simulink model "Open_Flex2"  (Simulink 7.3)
settings: Solver=ode4  StartTime=0.0  StopTime=20  RelTol=1e-3
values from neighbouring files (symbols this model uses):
  Ts = 0.04    [run.m]    (also in z2s_transf.m)
undefined symbols (not defined in the file or in its folder): Alfc, Apfc, Azpl, Blfc, Bpfc, Bzpl, Clfc, Cpfc, Czpl, Dlfc, Dpfc, Dzpl, TVC

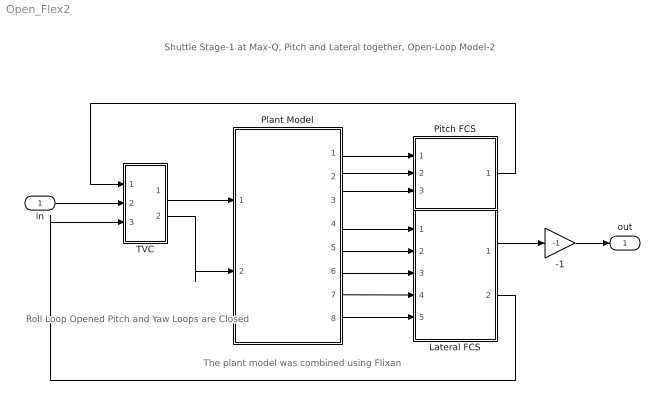
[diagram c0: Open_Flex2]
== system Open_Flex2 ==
  note: Shuttle Stage-1 at Max-Q, Pitch and Lateral together, Open-Loop Model-2
  note: Roll Loop Opened Pitch and Yaw Loops are Closed
  note: The plant model was combined using Flixan
  in : Inport  OutDataType=sfix(16)  OutScaling=2^0
  -1 : Gain  Gain=-1  ParameterDataType=sfix(16)  ParameterScaling=2^0  OutDataType=sfix(16)  OutScaling=2^0
  Lateral FCS : Subsystem
  Pitch FCS : Subsystem
  Plant Model : Subsystem
  TVC : Subsystem
  out : Outport  OutDataType=sfix(16)  OutScaling=2^0
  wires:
  TVC/1(dy) -> Plant Model/1(dy)
  TVC/2(dz) -> Plant Model/2(dz)
  -1/1 -> out/1
  Plant Model/8(Ny) -> Lateral FCS/5(Ny)
  Plant Model/7(r-flx) -> Lateral FCS/4(r)
  Plant Model/6(p-flx) -> Lateral FCS/3(p)
  Plant Model/5(psi) -> Lateral FCS/2(psi-er)
  Plant Model/4(phi) -> Lateral FCS/1(phi-er)
  Plant Model/3(Nz) -> Pitch FCS/3(Nz)
  Plant Model/2(q-flx) -> Pitch FCS/2(q)
  Plant Model/1(theta) -> Pitch FCS/1(theta)
  in/1 -> TVC/2(roll)
  Lateral FCS/1(DP_TVC) -> -1/1
  Pitch FCS/1(DQ_TVC) -> TVC/1(ptch)
  Lateral FCS/2(DR_TVC) -> TVC/3(yaw)

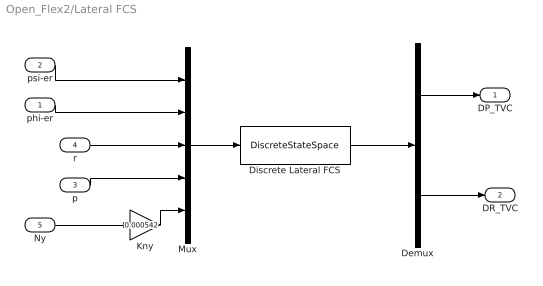
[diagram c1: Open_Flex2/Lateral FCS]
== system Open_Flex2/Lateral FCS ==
  phi-er : Inport  OutDataType=sfix(16)  OutScaling=2^0
  psi-er : Inport  Port=2  OutDataType=sfix(16)  OutScaling=2^0
  p : Inport  Port=3  OutDataType=sfix(16)  OutScaling=2^0
  r : Inport  Port=4  OutDataType=sfix(16)  OutScaling=2^0
  Ny : Inport  Port=5  OutDataType=sfix(16)  OutScaling=2^0
  Demux : Demux  Outputs=2
  Discrete Lateral FCS : DiscreteStateSpace  A=Alfc  B=Blfc  C=Clfc  D=Dlfc  SampleTime=Ts
  Kny : Gain  Gain=0.000542  ParameterDataType=sfix(16)  ParameterScaling=2^0  OutDataType=sfix(16)  OutScaling=2^0
  Mux : Mux  Inputs=5
  DP_TVC : Outport  OutDataType=sfix(16)  OutScaling=2^0
  DR_TVC : Outport  Port=2  OutDataType=sfix(16)  OutScaling=2^0
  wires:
  psi-er/1 -> Mux/1
  phi-er/1 -> Mux/2
  r/1 -> Mux/3
  Mux/1 -> Discrete Lateral FCS/1
  Discrete Lateral FCS/1 -> Demux/1
  Demux/1 -> DP_TVC/1
  Demux/2 -> DR_TVC/1
  p/1 -> Mux/4
  Ny/1 -> Kny/1
  Kny/1 -> Mux/5

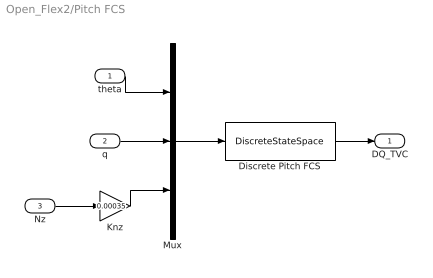
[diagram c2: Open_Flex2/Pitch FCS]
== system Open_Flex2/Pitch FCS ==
  theta : Inport  OutDataType=sfix(16)  OutScaling=2^0
  q : Inport  Port=2  OutDataType=sfix(16)  OutScaling=2^0
  Nz : Inport  Port=3  OutDataType=sfix(16)  OutScaling=2^0
  Discrete Pitch FCS : DiscreteStateSpace  A=Apfc  B=Bpfc  C=Cpfc  D=Dpfc  SampleTime=Ts
  Knz : Gain  Gain=0.00035  ParameterDataType=sfix(16)  ParameterScaling=2^0  OutDataType=sfix(16)  OutScaling=2^0
  Mux : Mux  Inputs=3
  DQ_TVC : Outport  OutDataType=sfix(16)  OutScaling=2^0
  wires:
  Mux/1 -> Discrete Pitch FCS/1
  Nz/1 -> Knz/1
  q/1 -> Mux/2
  theta/1 -> Mux/1
  Discrete Pitch FCS/1 -> DQ_TVC/1
  Knz/1 -> Mux/3

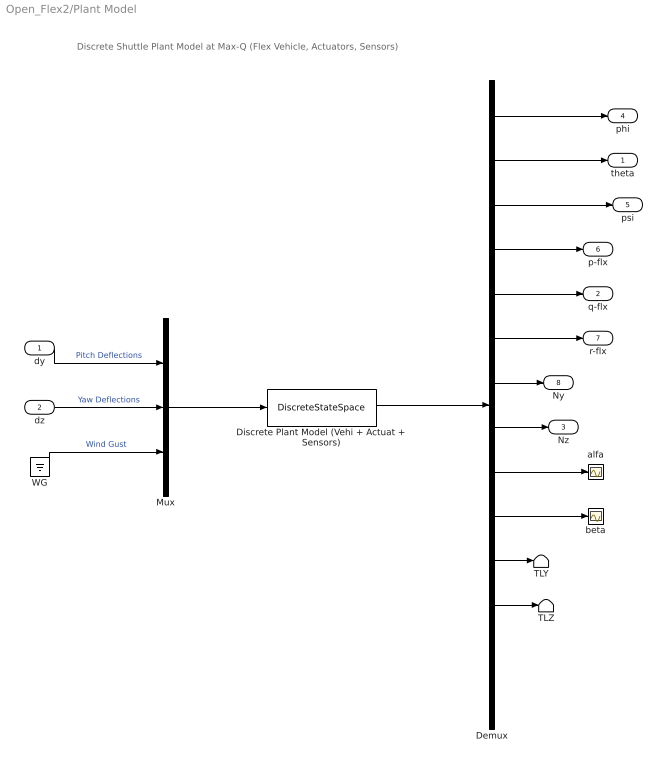
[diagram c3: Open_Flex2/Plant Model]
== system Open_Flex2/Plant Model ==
  note: Discrete Shuttle Plant Model at Max-Q (Flex Vehicle, Actuators, Sensors)
  dy : Inport  PortDimensions=5  OutDataType=sfix(16)  OutScaling=2^0
  dz : Inport  Port=2  PortDimensions=5  OutDataType=sfix(16)  OutScaling=2^0
  Demux : Demux  Outputs=[1,1,1,1,1,1,1,1,1,1, 5,5,5,5]
  Discrete Plant Model (Vehi + Actuat + Sensors) : DiscreteStateSpace  A=Azpl  B=Bzpl  C=Czpl  D=Dzpl  SampleTime=Ts
  Mux : Mux  Inputs="[5  5  1]"
  TLY : Terminator
  TLZ : Terminator
  WG : Ground
  alfa : Scope
  beta : Scope
  theta : Outport  OutDataType=sfix(16)  OutScaling=2^0
  q-flx : Outport  Port=2  OutDataType=sfix(16)  OutScaling=2^0
  Nz : Outport  Port=3  OutDataType=sfix(16)  OutScaling=2^0
  phi : Outport  Port=4  OutDataType=sfix(16)  OutScaling=2^0
  psi : Outport  Port=5  OutDataType=sfix(16)  OutScaling=2^0
  p-flx : Outport  Port=6  OutDataType=sfix(16)  OutScaling=2^0
  r-flx : Outport  Port=7  OutDataType=sfix(16)  OutScaling=2^0
  Ny : Outport  Port=8  OutDataType=sfix(16)  OutScaling=2^0
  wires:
  dy/1 -> Mux/1  "Pitch Deflections"
  dz/1 -> Mux/2  "Yaw Deflections"
  WG/1 -> Mux/3  "Wind Gust"
  Mux/1 -> Discrete Plant Model (Vehi + Actuat + Sensors)/1
  Discrete Plant Model (Vehi + Actuat + Sensors)/1 -> Demux/1
  Demux/1 -> phi/1
  Demux/2 -> theta/1
  Demux/3 -> psi/1
  Demux/4 -> p-flx/1
  Demux/5 -> q-flx/1
  Demux/6 -> r-flx/1
  Demux/7 -> Ny/1
  Demux/8 -> Nz/1
  Demux/9 -> alfa/1
  Demux/10 -> beta/1
  Demux/11 -> TLY/1
  Demux/12 -> TLZ/1

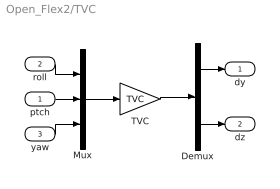
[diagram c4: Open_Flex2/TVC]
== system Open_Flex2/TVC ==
  ptch : Inport  OutDataType=sfix(16)  OutScaling=2^0
  roll : Inport  Port=2  OutDataType=sfix(16)  OutScaling=2^0
  yaw : Inport  Port=3  OutDataType=sfix(16)  OutScaling=2^0
  Demux : Demux  Outputs="[5  5]"
  Mux : Mux  Inputs=3
  TVC : Gain  Gain=TVC  Multiplication=Matrix(K*u) (u vector)  ParameterDataType=sfix(16)  ParameterScaling=2^0  OutDataType=sfix(16)  OutScaling=2^0
  dy : Outport  OutDataType=sfix(16)  OutScaling=2^0
  dz : Outport  Port=2  OutDataType=sfix(16)  OutScaling=2^0
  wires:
  TVC/1 -> Demux/1
  Mux/1 -> TVC/1
  roll/1 -> Mux/1
  Demux/1 -> dy/1
  ptch/1 -> Mux/2
  Demux/2 -> dz/1
  yaw/1 -> Mux/3
